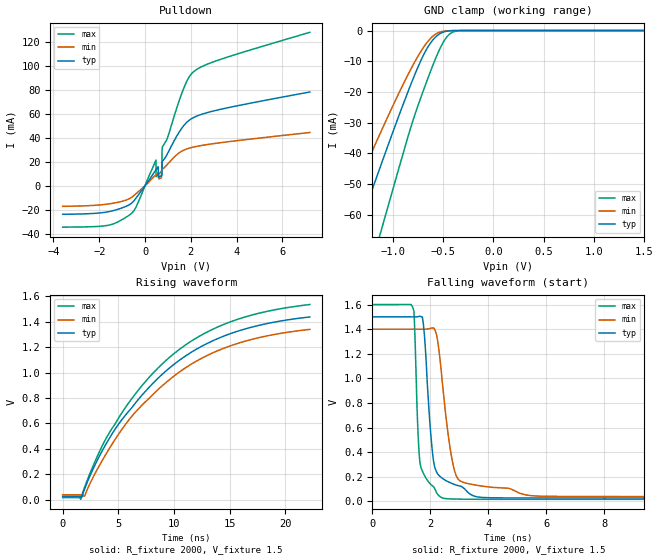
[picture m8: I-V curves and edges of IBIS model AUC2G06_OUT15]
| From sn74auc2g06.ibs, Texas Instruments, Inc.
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[Model]   AUC2G06_OUT15
Model_type  Open_drain
Enable   Active-Low
Vref =   0
Rref =   2000
Cref =   15p
Vmeas =   0.75
| variable   typ   min   max
C_comp   3.01pF   2.60pF   3.26pF
| C_pulldown   4.79pF   1.98pF   12.89pF
| C_tri-state   3.01pF   2.60pF   3.26pF
[Temperature Range]   40   100   -40
| Ambient temperature   25   85   -40
[Voltage range]   1.5   1.4   1.6
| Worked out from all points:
|   slope of the pulldown table from 0 to 0.225 V, typ, clamps not added: 37.3 ohm
|   GND clamp passes 1 mA (typ) near -0.53 V on its own axis
|   rising waveform, R_fixture 2000, V_fixture 1.5: 20-80 % time 8.37ns typ, 8.32ns min, 8.28ns max; typ from 0.027 V to 1.44 V
|   falling waveform, R_fixture 2000, V_fixture 1.5: 20-80 % time 277ps typ, 426ps min, 157ps max; typ from 1.5 V to 0.027 V
[GND Clamp]
| AUC2G06_OUT15
|   Voltage   I(typ)   I(min)   I(max)
-3.6V     -279.3mA   -228.7mA   -348mA
-1.535V   -82.96mA   -64.34mA   -113.9mA
-1.35V    -65.56mA   -50.29mA   -92.6mA
-1.15V    -46.98mA   -35.46mA   -69.44mA
-1.1V     -42.39mA   -31.84mA   -63.64mA
-825mV    -18.08mA   -12.98mA   -32.18mA
-685mV    -7.459mA   -5.101mA   -18.71mA
-560mV    -1.73mA    -927.3uA   -8.105mA
-495mV    -497.5uA   -233uA     -3.727mA
-430mV    -100.1uA   -51.64uA   -1.068mA
-305mV    -2.545uA   -2.096uA   -19.74uA
1.5V      322pA      494.6pA    331.6pA
[Pulldown]
| AUC2G06_OUT15
|   Voltage   I(typ)   I(min)   I(max)
-3.6V     -23.87mA   -17.26mA   -34.61mA
-1.565V   -21.6mA    -15.16mA   -32.85mA
-520mV    -13.36mA   -8.764mA   -21.72mA
480mV     13.33mA    9.224mA    21.44mA
485mV     13.46mA    9.315mA    7.619mA
720mV     8.537mA    6.727mA    11.81mA
735mV     8.725mA    13.39mA    12.06mA
745mV     18.83mA    13.54mA    29.66mA
760mV     20.34mA    13.77mA    32.32mA
1.73V     50.99mA    29.95mA    83.08mA
2.16V     57.23mA    32.4mA     95.69mA
7.2V      78.2mA     44.4mA     128mA
[Ramp]
| AUC2G06_OUT15
| variable   typ   min   max
dV/dt_r   0.85/8.38E-09   0.79/8.33E-09   0.92/8.28E-09
dV/dt_f   0.89/2.84E-10   0.82/4.35E-10   0.95/1.67E-10
R_load = 2000
[Rising Waveform]
| AUC2G06_OUT15
R_fixture =   2000
C_fixture =   0
L_fixture =   0
V_fixture =   1.5
V_fixture_min = 1.4
V_fixture_max = 1.6
|   Time   V(typ)   V(min)   V(max)
0s        27.17mV    38.78mV    16.4mV
1.625ns   24.17mV    38.71mV    2.956mV
1.985ns   87.43mV    31.64mV    101.1mV
3.42ns    362.9mV    287.5mV    399.7mV
5.33ns    631mV      554.8mV    685.3mV
7.715ns   879.7mV    793.3mV    958.1mV
10.24ns   1.082V     989.3mV    1.167V
12.63ns   1.214V     1.12V      1.304V
15.34ns   1.315V     1.219V     1.408V
22.2ns    1.438V     1.341V     1.536V
[Falling Waveform]
| AUC2G06_OUT15
R_fixture =   2000
C_fixture =   0
L_fixture =   0
V_fixture =   1.5
V_fixture_min = 1.4
V_fixture_max = 1.6
|   Time   V(typ)   V(min)   V(max)
0s        1.5V       1.4V       1.6V
1.425ns   1.5V       1.4V       1.554V
1.59ns    1.503V     1.4V       476.9mV
1.72ns    1.498V     1.4V       248.2mV
2.1ns     343.9mV    1.411V     121.1mV
2.445ns   182mV      894mV      25.72mV
2.725ns   147.3mV    369.7mV    19.59mV
2.97ns    127.5mV    177.6mV    18.14mV
5.3ns     27.32mV    51.85mV    16.41mV
22.2ns    27.17mV    38.78mV    16.4mV
